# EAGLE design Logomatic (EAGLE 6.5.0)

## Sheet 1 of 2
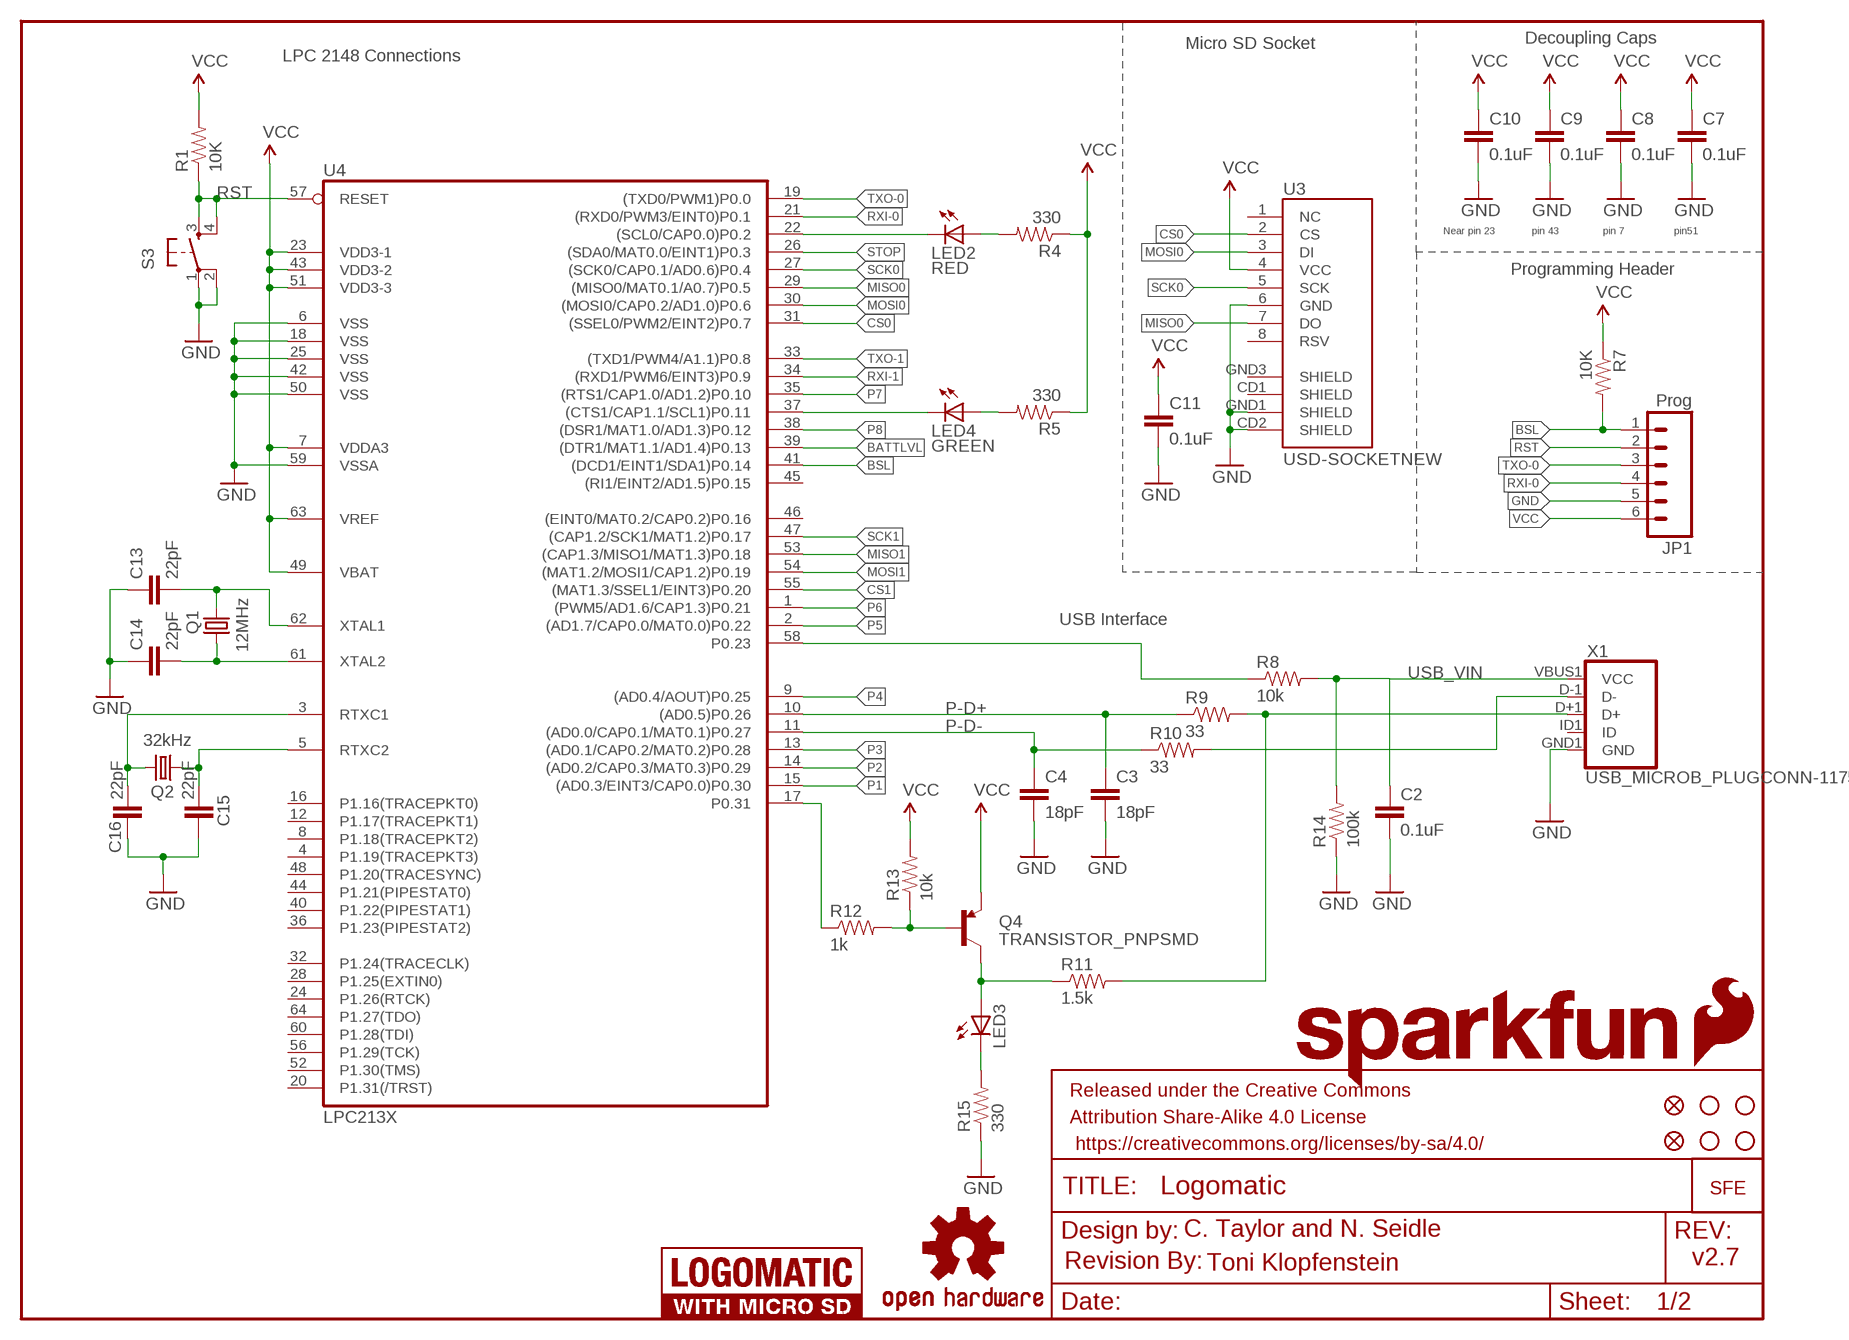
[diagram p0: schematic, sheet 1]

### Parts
C2  0.1uF  0.1UF-25V(+80/-20%)(0603)  [0603-CAP]
C3  18pF  18PF-50V-5%(0603)  [0603-CAP]
C4  18pF  18PF-50V-5%(0603)  [0603-CAP]
C7  0.1uF  0.1UF-25V(+80/-20%)(0603)  [0603-CAP]
C8  0.1uF  0.1UF-25V(+80/-20%)(0603)  [0603-CAP]
C9  0.1uF  0.1UF-25V(+80/-20%)(0603)  [0603-CAP]
C10  0.1uF  0.1UF-25V(+80/-20%)(0603)  [0603-CAP]
C11  0.1uF  0.1UF-25V(+80/-20%)(0603)  [0603-CAP]
C13  22pF  22PF-50V-5%(0603)  [0603-CAP]
C14  22pF  22PF-50V-5%(0603)  [0603-CAP]
C15  22pF  22PF-50V-5%(0603)  [0603-CAP]
C16  22pF  22PF-50V-5%(0603)  [0603-CAP]
FRAME2  FRAME-LETTER  [CREATIVE_COMMONS]
JP1  Prog  M06SIP  [1X06]
LED2  RED  LED-RED0603  [LED-0603]
LED3  LED-RED0603  [LED-0603]
LED4  GREEN  LED-GREEN0603  [LED-0603]
LOGO1  OSHW-LOGOL  [OSHW-LOGO-L]
LOGO2  SFE_LOGO_NAME.1_INCH  [SFE_LOGO_NAME_.1]
LOGO3  SFE_LOGO_FLAME.4_INCH  [SFE_LOGO_FLAME_.4]
Q1  12MHz  CRYSTAL5X3  [CRYSTAL-SMD-5X3]
Q2  32kHz  CRYSTAL32-SMD  [CRYSTAL-32KHZ-SMD]
Q4  TRANSISTOR_PNPSMD  [SOT23-3]
R1  10K  10KOHM1/10W1%(0603)0603  [0603-RES]
R4  330  330OHM1/10W1%(0603)  [0603-RES]
R5  330  330OHM1/10W1%(0603)  [0603-RES]
R7  10K  10KOHM1/10W1%(0603)0603  [0603-RES]
R8  10k  10KOHM1/10W1%(0603)0603  [0603-RES]
R9  33  33OHM1/10W1%(0603)  [0603]
R10  33  33OHM1/10W1%(0603)  [0603]
R11  1.5k  1.5KOHM1/10W1%(0603)  [0603]
R12  1k  1KOHM1/10W1%(0603)  [0603-RES]
R13  10k  10KOHM1/10W1%(0603)0603  [0603-RES]
R14  100k  100KOHM1/10W1%(0603)  [0603-RES]
R15  330  330OHM1/10W1%(0603)  [0603-RES]
S3  Reset  TAC_SWITCHSND  [TACTILE_SWITCH_SMD]
U3  USD-SOCKETNEW  [MICRO-SD-SOCKET-PP]
U4  LPC213X  [SQFP-S-10X10-64]
U$1  FIDUCIAL1X2  [FIDUCIAL-1X2]
U$2  FIDUCIAL1X2  [FIDUCIAL-1X2]
U$3  STAND-OFF  [STAND-OFF]
U$4  STAND-OFF  [STAND-OFF]
U$5  STAND-OFF  [STAND-OFF]
U$6  LOGOMATIC_LOGO  [LOGOMATIC_LOGO]
U$7  LOGO-SFESK  [SFE-LOGO-FLAME]
U$8  STAND-OFF  [STAND-OFF]
U$10  REVISION  [REVISION]
X1  USB_MICROB_PLUGCONN-11752  [USB-B-MICRO-SMD_V03]

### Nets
BATTLVL: U4.39((DTR1/MAT1.1/AD1.4)P0.13) ; also sheet 2
BSL: JP1.1 R7.2 U4.41((DCD1/EINT1/SDA1)P0.14)
CS0: U3.2(CS) U4.31((SSEL0/PWM2/EINT2)P0.7)
CS1: U4.55((MAT1.3/SSEL1/EINT3)P0.20) ; also sheet 2
GND [power]: C2.2 C3.2 C4.2 C7.2 C8.2 C9.2 C10.2 C11.2 C13.1 C14.1 C15.1 C16.1 JP1.5 R14.1 R15.1 S3.1 S3.2 U3.6(GND) U3.CD2(SHIELD) U3.GND1(SHIELD) U4.6(VSS) U4.18(VSS) U4.25(VSS) U4.42(VSS) U4.50(VSS) U4.59(VSSA) X1.GND1(GND) ; also sheet 2
MISO0: U3.7(DO) U4.29((MISO0/MAT0.1/A0.7)P0.5)
MISO1: U4.53((CAP1.3/MISO1/MAT1.3)P0.18) ; also sheet 2
MOSI0: U3.3(DI) U4.30((MOSI0/CAP0.2/AD1.0)P0.6)
MOSI1: U4.54((MAT1.2/MOSI1/CAP1.2)P0.19) ; also sheet 2
N$5: C13.2 Q1.3 U4.62(XTAL1)
N$6: C16.2 Q2.X2 U4.3(RTXC1)
N$7: LED2.A R4.2
N$9: C15.2 Q2.X1 U4.5(RTXC2)
N$16: R8.1 U4.58(P0.23)
N$17: Q4.1(B) R12.2 R13.1
N$19: LED4.A R5.2
N$21: C14.2 Q1.1 U4.61(XTAL2)
N$31: R12.1 U4.17(P0.31)
N$33: LED3.C R15.2
P1: U4.15((AD0.3/EINT3/CAP0.0)P0.30) ; also sheet 2
P2: U4.14((AD0.2/CAP0.3/MAT0.3)P0.29) ; also sheet 2
P3: U4.13((AD0.1/CAP0.2/MAT0.2)P0.28) ; also sheet 2
P4: U4.9((AD0.4/AOUT)P0.25) ; also sheet 2
P5: U4.2((AD1.7/CAP0.0/MAT0.0)P0.22) ; also sheet 2
P6: U4.1((PWM5/AD1.6/CAP1.3)P0.21) ; also sheet 2
P7: U4.35((RTS1/CAP1.0/AD1.2)P0.10) ; also sheet 2
P8: U4.38((DSR1/MAT1.0/AD1.3)P0.12) ; also sheet 2
P-D+: C3.1 R9.1 U4.10((AD0.5)P0.26)
P-D-: C4.1 R10.1 U4.11((AD0.0/CAP0.1/MAT0.1)P0.27)
RST: JP1.2 R1.1 S3.3 S3.4 U4.57(RESET)
RXI-0: JP1.4 U4.21((RXD0/PWM3/EINT0)P0.1)
RXI-1: U4.34((RXD1/PWM6/EINT3)P0.9) ; also sheet 2
SCK0: U3.5(SCK) U4.27((SCK0/CAP0.1/AD0.6)P0.4)
SCK1: U4.47((CAP1.2/SCK1/MAT1.2)P0.17) ; also sheet 2
STAT: LED3.A Q4.3(C) R11.1
STAT0: LED2.C U4.22((SCL0/CAP0.0)P0.2)
STAT1: LED4.C U4.37((CTS1/CAP1.1/SCL1)P0.11)
STOP: U4.26((SDA0/MAT0.0/EINT1)P0.3) ; also sheet 2
TXO-0: JP1.3 U4.19((TXD0/PWM1)P0.0)
TXO-1: U4.33((TXD1/PWM4/A1.1)P0.8) ; also sheet 2
USB_D+: R9.2 R11.2 X1.D+1(D+)
USB_D-: R10.2 X1.D-1(D-)
USB_VIN: C2.1 R8.2 R14.2 X1.VBUS1(VCC) ; also sheet 2
VCC: C7.1 C8.1 C9.1 C10.1 C11.1 JP1.6 Q4.2(E) R1.2 R4.1 R5.1 R7.1 R13.2 U3.4(VCC) U4.7(VDDA3) U4.23(VDD3-1) U4.43(VDD3-2) U4.49(VBAT) U4.51(VDD3-3) U4.63(VREF) ; also sheet 2
Unconnected: U3.1(NC) U3.8(RSV) U3.CD1(SHIELD) U3.GND3(SHIELD) U4.4(P1.19(TRACEPKT3)) U4.8(P1.18(TRACEPKT2)) U4.12(P1.17(TRACEPKT1)) U4.16(P1.16(TRACEPKT0)) U4.20(P1.31(/TRST)) U4.24(P1.26(RTCK)) U4.28(P1.25(EXTIN0)) U4.32(P1.24(TRACECLK)) U4.36(P1.23(PIPESTAT2)) U4.40(P1.22(PIPESTAT1)) U4.44(P1.21(PIPESTAT0)) U4.45((RI1/EINT2/AD1.5)P0.15) U4.46((EINT0/MAT0.2/CAP0.2)P0.16) U4.48(P1.20(TRACESYNC)) U4.52(P1.30(TMS)) U4.56(P1.29(TCK)) U4.60(P1.28(TDI)) U4.64(P1.27(TDO)) X1.ID1(ID)

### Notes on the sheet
- Decoupling Caps
- Micro SD Socket
- LPC 2148 Connections
- Near pin 23 | pin 43 | pin 7 | pin51
- Programming Header
- USB Interface
- C. Taylor and N. Seidle
- Toni Klopfenstein | v2.7

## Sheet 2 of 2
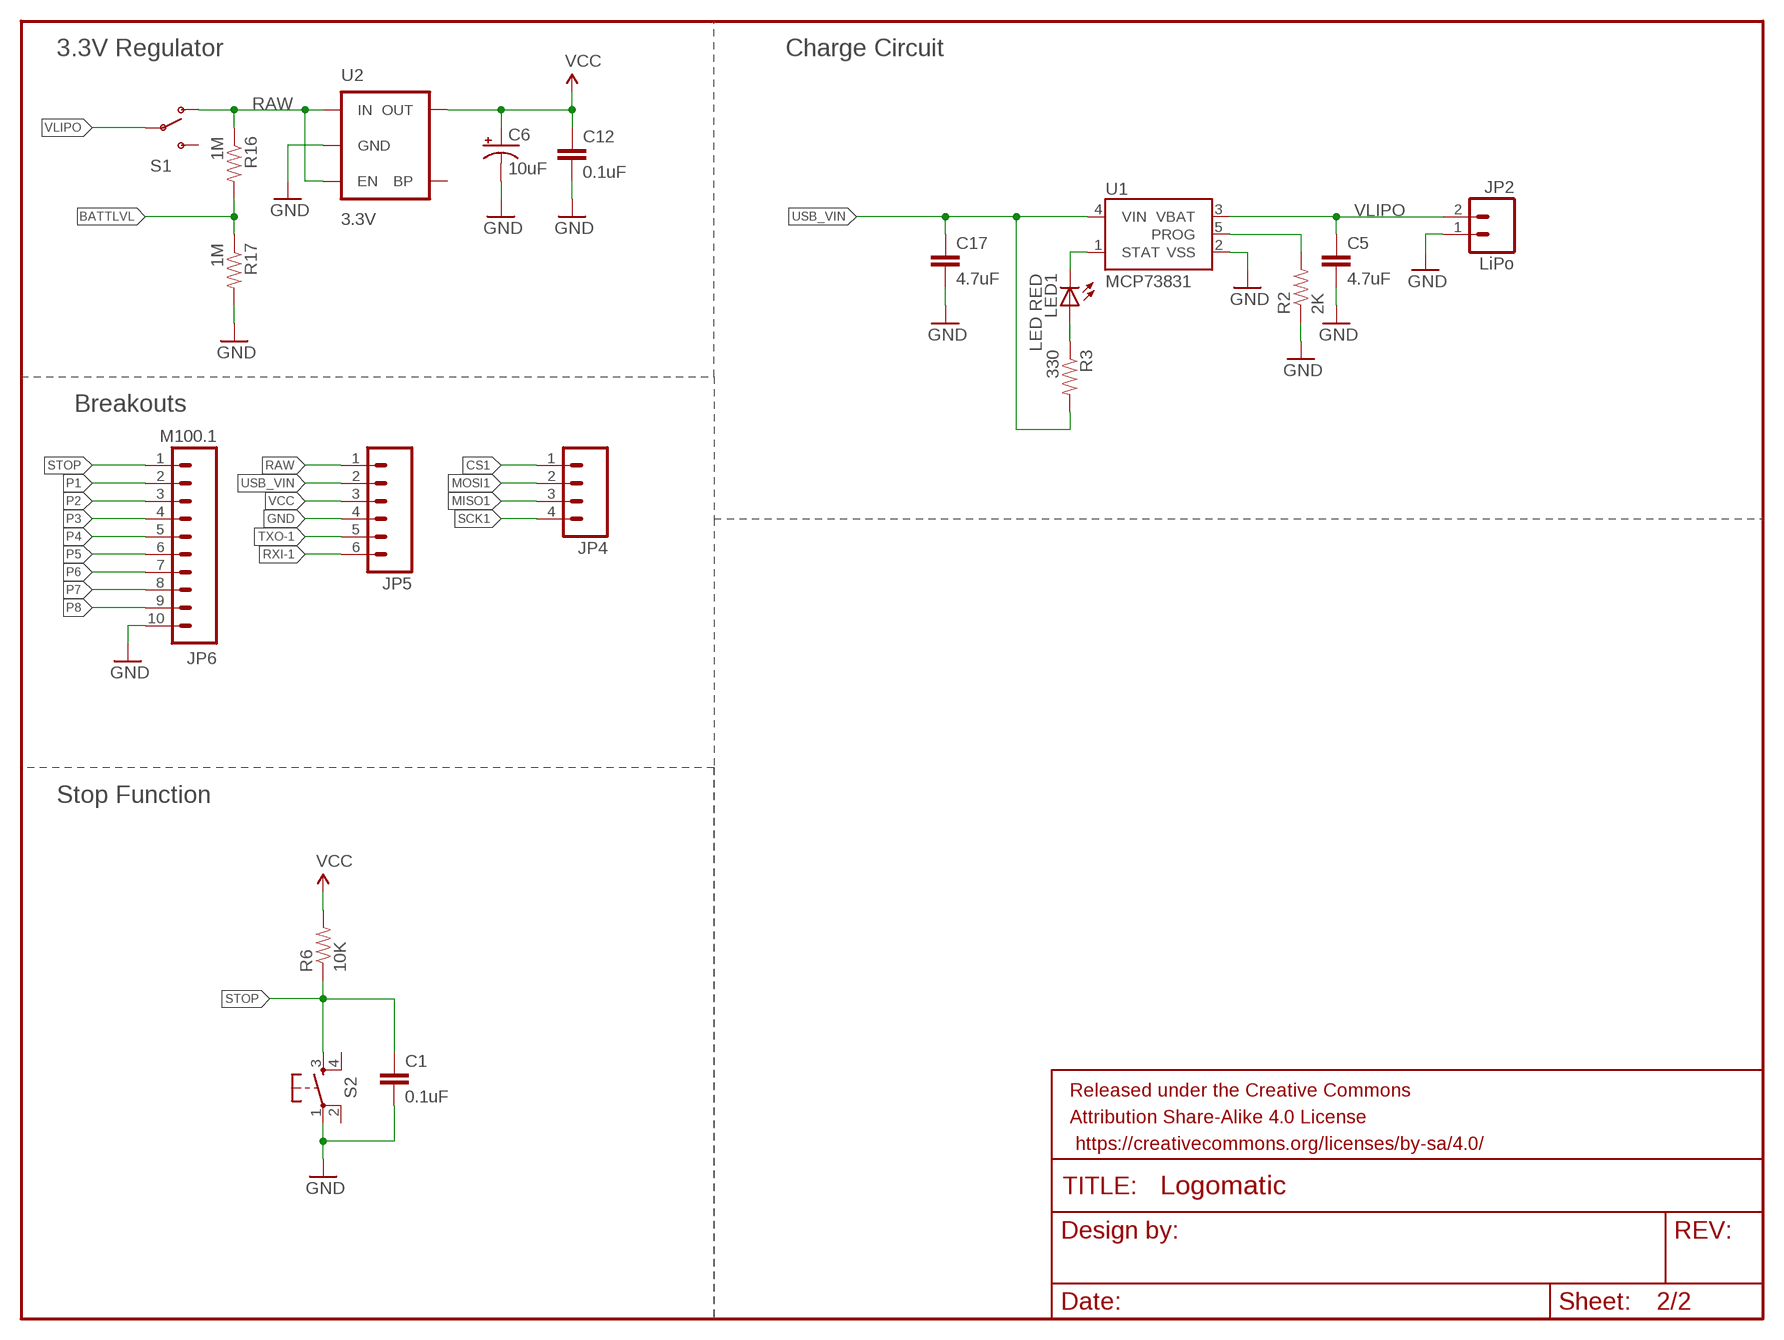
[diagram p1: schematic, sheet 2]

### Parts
C1  0.1uF  0.1UF-25V(+80/-20%)(0603)  [0603-CAP]
C5  4.7uF  4.7UF-6.3V-10%(0603)0603  [0603-CAP]
C6  10uF  10UF-16V-10%(TANT)  [EIA3216]
C12  0.1uF  0.1UF-25V(+80/-20%)(0603)  [0603-CAP]
C17  4.7uF  4.7UF-6.3V-10%(0603)0603  [0603-CAP]
FRAME4  FRAME-LETTER  [CREATIVE_COMMONS]
JP2  LiPo  M02-JST-2MM-SMT  [JST-2-SMD]
JP4  M04PTH  [1X04]
JP5  M06SIP  [1X06]
JP6  M100.1  M10"  [1X10]
LED1  LED RED  LED-RED0603  [LED-0603]
R2  2K  2.0KOHM1/10W5%(0603)  [0603-RES]
R3  330  330OHM1/10W1%(0603)  [0603-RES]
R6  10K  10KOHM1/10W1%(0603)0603  [0603-RES]
R16  1M  1MOHM1/10W1%(0603)  [0603-RES]
R17  1M  1MOHM1/10W1%(0603)  [0603-RES]
S1  SWITCH-SPSTSMD  [AYZ0202]
S2  Stop  TAC_SWITCHSND  [TACTILE_SWITCH_SMD]
U1  MCP73831  MCP73831SMD  [SOT23-5]
U2  3.3V  V_REG_LDOSMD  [SOT23-5]

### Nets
BATTLVL: R16.2 R17.1 ; also sheet 1
CS1: JP4.1 ; also sheet 1
GND [power]: C1.2 C5.2 C6.C(-) C12.2 C17.2 JP2.1 JP5.4 JP6.10 R2.1 R17.2 S2.1 U1.2(VSS) U2.2(GND) ; also sheet 1
MISO1: JP4.3 ; also sheet 1
MOSI1: JP4.2 ; also sheet 1
N$1: R2.2 U1.5(PROG)
N$12: LED1.C U1.1(STAT)
N$13: LED1.A R3.1
P1: JP6.2 ; also sheet 1
P2: JP6.3 ; also sheet 1
P3: JP6.4 ; also sheet 1
P4: JP6.5 ; also sheet 1
P5: JP6.6 ; also sheet 1
P6: JP6.7 ; also sheet 1
P7: JP6.8 ; also sheet 1
P8: JP6.9 ; also sheet 1
RAW: JP5.1 R16.1 S1.1(O) U2.1(IN) U2.3(EN)
RXI-1: JP5.6 ; also sheet 1
SCK1: JP4.4 ; also sheet 1
STOP: C1.1 JP6.1 R6.1 S2.3 ; also sheet 1
TXO-1: JP5.5 ; also sheet 1
USB_VIN: C17.1 JP5.2 R3.2 U1.4(VIN) ; also sheet 1
VCC: C6.A(+) C12.1 JP5.3 R6.2 U2.5(OUT) ; also sheet 1
VLIPO [power]: C5.1 JP2.2 S1.2(P) U1.3(VBAT)
Unconnected: S1.3(S) S2.2 S2.4 U2.4(BP)

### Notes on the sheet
- 3.3V Regulator | Charge Circuit
- Breakouts
- Stop Function

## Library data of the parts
C1 C2 C7-C12 = SparkFun-Capacitors:0.1UF-25V(+80/-20%)(0603): CAP-00810; PROD_ID: CAP-00810
C3 C4 = SparkFun-Capacitors:18PF-50V-5%(0603): CAP-08267; PROD_ID: CAP-08267
C5 C17 = SparkFun-Capacitors:4.7UF-6.3V-10%(0603): CAP-08280; PROD_ID: CAP-08280
C6 = SparkFun-Capacitors:10UF-16V-10%(TANT): CAP-00811; PROD_ID: CAP-00811
C13-C16 = SparkFun-Capacitors:22PF-50V-5%(0603): CAP-07876; PROD_ID: CAP-07876
FRAME2 FRAME4 = SparkFun-Aesthetics:FRAME-LETTER: Schematic Frame
JP1 JP5 = SparkFun:M06: Header 6 Standard 6-pin 0.1" header. Use with straight break away headers (SKU : PRT-00116), right angle break away headers (PRT-00553), swiss pins (PRT-00743), machine pins (PRT-00117), and female headers (PRT-00115). Molex polarized connector foot print use with SKU : PRT-08094 with associated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
JP2 = SparkFun:M02: Header 2
JP4 = SparkFun:M04: Header 4 Standard 4-pin 0.1" header. Use with straight break away headers (SKU : PRT-00116), right angle break away headers (PRT-00553), swiss pins (PRT-00743), machine pins (PRT-00117), and female headers (PRT-00115). Molex polarized connector foot print use with SKU : PRT-08231 with associated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
JP6 = SparkFun:M10: Header 10 Standard 10-pin 0.1" header. Use with straight break away headers (SKU : PRT-00116), right angle break away headers (PRT-00553), swiss pins (PRT-00743), machine pins (PRT-00117), and female headers (PRT-00115).
LED1 LED3 = SparkFun-LED:LED-RED: Assorted Red LEDs; PROD_ID: DIO-00819; VALUE: RED
LED2 = SparkFun-LED:LED-RED: Assorted Red LEDs; PROD_ID: DIO-00819
LED4 = SparkFun-LED:LED-GREEN: Various green LEDs; PROD_ID: DIO-00821
LOGO1 = SparkFun-Aesthetics:OSHW-LOGO: Open Source Hardware Logo This logo indicates the piece of hardware it is found on incorporates a OSHW license and/or adheres to the definition of open source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
LOGO2 = SparkFun-Aesthetics:SFE_LOGO_NAME: SFE Logo, name only
LOGO3 = SparkFun-Aesthetics:SFE_LOGO_FLAME: SFE Logo, flame only
Q1 = SparkFunEagle-6-6-07:CRYSTAL: Crystals
Q2 = SparkFun:CRYSTAL: Crystals
Q4 = SparkFun:TRANSISTOR_PNP
R1 R6 R7 = SparkFun-Resistors:10KOHM1/10W1%(0603): RES-00824; PROD_ID: RES-00824
R2 = SparkFun-Resistors:2.0KOHM1/10W5%(0603): RES-08296; PROD_ID: RES-08296; VALUE: 2.0k
R3-R5 R15 = SparkFun-Resistors:330OHM1/10W1%(0603): RES-00818; PROD_ID: RES-00818
R8 R13 = SparkFun-Resistors:10KOHM1/10W1%(0603): RES-00824; PROD_ID: RES-00824; VALUE: 10K
R9 R10 = SparkFun-Resistors:33OHM1/10W1%(0603): RES-08270; PROD_ID: RES-08270; VALUE: 33OHM
R11 = SparkFun-Resistors:1.5KOHM1/10W1%(0603): RES-08306; PROD_ID: RES-08306; VALUE: 1.5KOHM
R12 = SparkFun-Resistors:1KOHM1/10W1%(0603): RES-07856; PROD_ID: RES-07856; VALUE: 1K
R14 = SparkFun-Resistors:100KOHM1/10W1%(0603): RES-07828; PROD_ID: RES-07828
R16 R17 = SparkFun-Resistors:1MOHM1/10W1%(0603): RES-07868; PROD_ID: RES-07868
S1 = SparkFun:SWITCH-SPST: SPST Switch Simple slide switch. Spark Fun Electronics SKU : COM-00102
S2 S3 = SparkFunEagle-6-6-07:TAC_SWITCH: Momentary Switch Button commonly used for reset or general input. Spark Fun Electronics SKU : COM-00097
U1 = SparkFun:MCP73831
U2 = SparkFun:V_REG_LDO: Voltage Regulator LDO Standard 150mA LDO voltage regulator in SOT-23 layout. Micrel part MIC5205. BP (by-pass) pin is used to lower output noise with 470pF cap.
U3 = SparkFun-Connectors:USD-SOCKET: microSD Socket Push-push type uSD socket. Schematic element and footprint production proven. Spark Fun Electronics SKU : PRT-00127. tDoc lines correctly indicate media card edge positions when inserting (unlocked, locked, depressed).
U4 = SparkFun:LPC213X: LPC213x Schematic element and footprint for NXP LPC213x. Spark Fun Electronics SKU : COM-00520
U$1 U$2 = SparkFun:FIDUCIAL: Fiducial Alignment Points
U$3-U$5 U$8 = SparkFun:STAND-OFF: Stand Off
U$6 = SparkFun-Aesthetics:LOGOMATIC_LOGO: Logo for the Logomatic boards.
U$7 = SparkFun:LOGO-SFE: Spark Fun Electronics PCB Logo
U$10 = SparkFun-Aesthetics:REVISION
X1 = SparkFun-Connectors:USB_MICROB_PLUG: USB Micro-B Plug Comes in a variety of packages. Check out Hirose's ZX-x0 line: http://www.hirose.co.jp/cataloge_hp/e24200011.pdf; PROD_ID: CONN-11752

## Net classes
0 default: width 0.178 mm
1 power: width 0.203 mm
2 hv: width 0.254 mm, clearance 0.229 mm

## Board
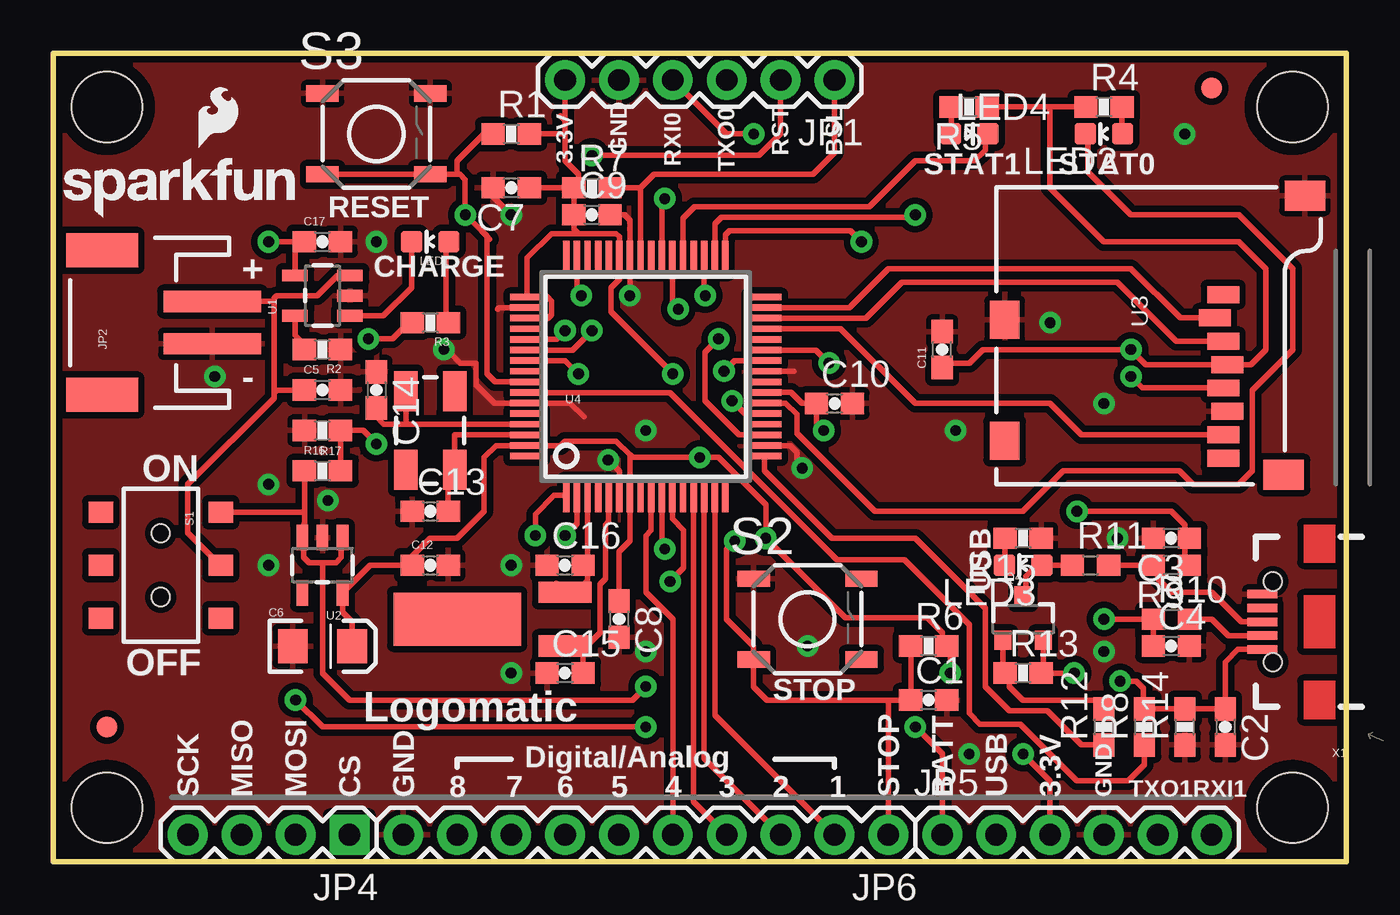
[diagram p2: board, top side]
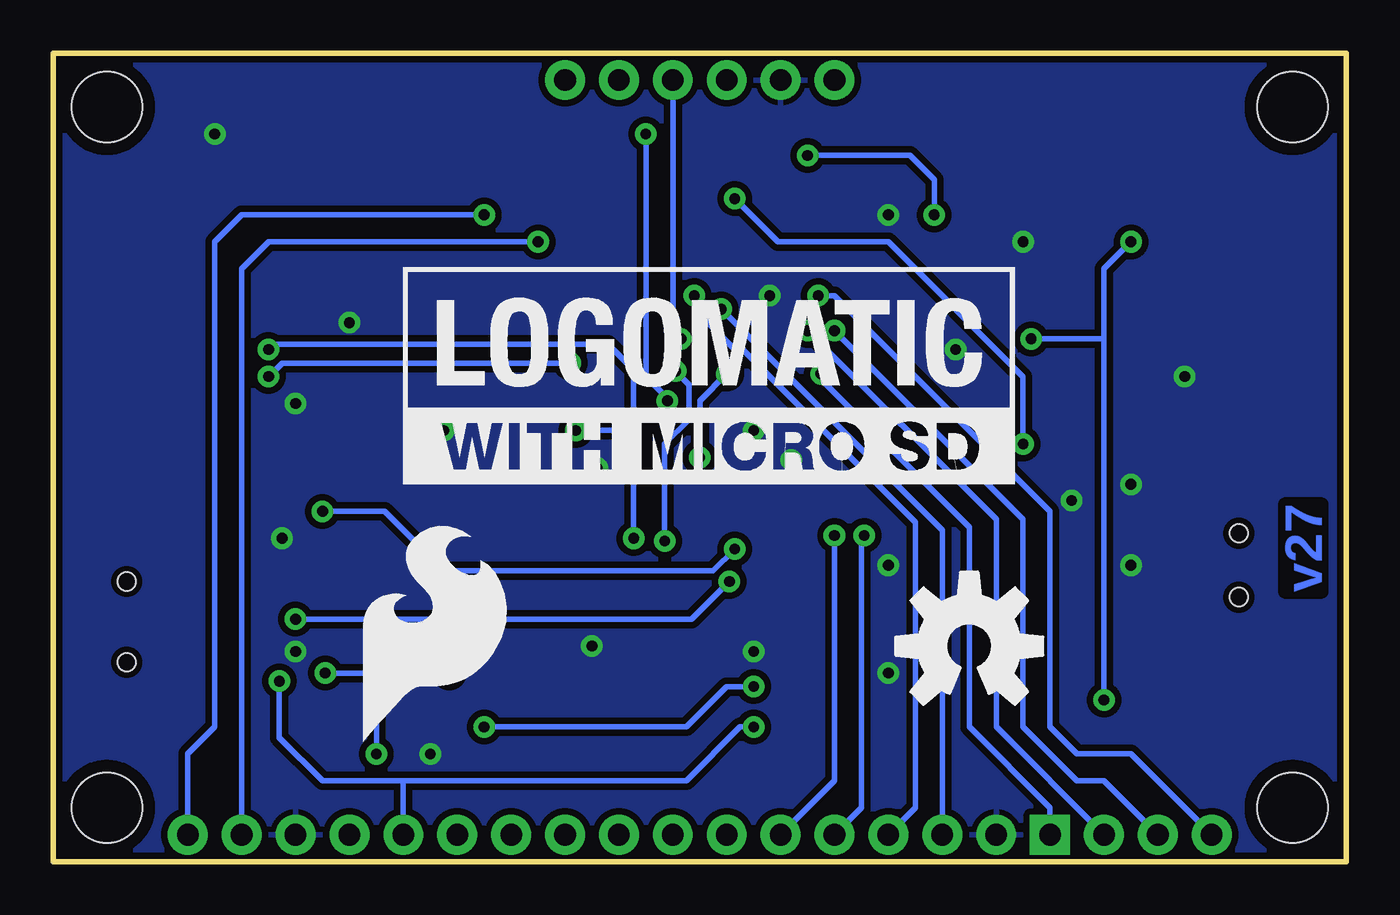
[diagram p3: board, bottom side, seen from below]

Size 60.96 x 38.1 mm. Coordinates in mm from the lower left corner, seen from the top.
Outline: 0,0 60.96,0 60.96,38.1 0,38.1 0,0
Copper layers (1*16): Top 0.035mm / dielectric 1.5mm / Bottom 0.035mm
Design rules "SparkFun *": minimum track width 8mil, minimum drill 20mil, track to track 8mil, track to pad 8mil, pad to pad 7mil, via to via 8mil, smd to smd 8mil, copper to edge 10mil, drill to drill 8mil, minimum pad ring 12mil, minimum via ring 10mil, stop-mask expansion 4mil, vias tented up to drill 20mil, thermal gap 10mil

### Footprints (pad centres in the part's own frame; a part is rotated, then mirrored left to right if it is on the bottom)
0603-CAP = smd 1.1 x 1: 1 -0.85,0; 2 0.85,0
EIA3216 = smd 1.4 x 1.6: A 1.4,0; C -1.4,0
1X06 = drill 1.016 pad 1.88: 1 0,0; 2 2.54,0; 3 5.08,0; 4 7.62,0; 5 10.16,0; 6 12.7,0
JST-2-SMD = smd 1 x 4.6: 1 -1,-3.7; 2 1,-3.7 | smd 1.6 x 3.4: NC1 -3.4,1.5; NC2 3.4,1.5
1X04 = drill 1.016 pad 1.88 square: 1 0,0 | drill 1.016 pad 1.88: 2 2.54,0; 3 5.08,0; 4 7.62,0
1X10 = drill 1.016 pad 1.88: 1 0,0; 2 2.54,0; 3 5.08,0; 4 7.62,0; 5 10.16,0; 6 12.7,0; 7 15.24,0; 8 17.78,0; 9 20.32,0; 10 22.86,0
LED-0603 = smd 1 x 1: A 0,-0.877; C 0,0.877
CRYSTAL-SMD-5X3 = smd 1.9 x 1.1: 1 -1.85,-1.15; 2 1.85,-1.15; 3 1.85,1.15; 4 -1.85,1.15
CRYSTAL-32KHZ-SMD = smd 2.5 x 6: SHEILD 0,5.08 | smd 1 x 2.5: X1 -1.27,0; X2 1.27,0
SOT23-3 = smd 0.8 x 0.9: 1 -0.95,-1; 2 0.95,-1; 3 0,1.1
0603-RES = smd 1.1 x 1: 1 -0.85,0; 2 0.85,0
0603 = smd 1.1 x 1: 1 -0.85,0; 2 0.85,0
AYZ0202 = smd 1 x 1.15: 1 -2.5,2.825; 2 0,2.825; 3 2.5,2.825; 4 -2.5,-2.825; 5 0,-2.825; 6 2.5,-2.825 | hole 0.85: 1.5,0; -1.5,0
TACTILE_SWITCH_SMD = smd 1.524 x 0.762: 1 -2.54,1.905; 2 2.54,1.905; 3 -2.54,-1.905; 4 2.54,-1.905
SOT23-5 = smd 0.55 x 1.2: 1 -0.95,-1.3; 2 0,-1.3; 3 0.95,-1.3; 4 0.95,1.3; 5 -0.95,1.3
MICRO-SD-SOCKET-PP = smd 0.8 x 1.5: 1 -8.94,10.7; 2 -7.84,10.3; 3 -6.74,10.7; 4 -5.64,10.9; 5 -4.54,10.7; 6 -3.44,10.9; 7 -2.34,10.7; 8 -1.24,10.7 | smd 1.8 x 1.4: CD1 -2.05,0.4; CD2 -7.75,0.4 | smd 1.4 x 1.9: GND1 -13.6,14.55; GND3 -0.45,13.55
SQFP-S-10X10-64 = smd 0.3 x 1.6: 1 -3.75,-5.6; 2 -3.25,-5.6; 3 -2.75,-5.6; 4 -2.25,-5.6; 5 -1.75,-5.6; 6 -1.25,-5.6; 7 -0.75,-5.6; 8 -0.25,-5.6; 9 0.25,-5.6; 10 0.75,-5.6; 11 1.25,-5.6; 12 1.75,-5.6; 13 2.25,-5.6; 14 2.75,-5.6; 15 3.25,-5.6; 16 3.75,-5.6; 33 3.75,5.6; 34 3.25,5.6; 35 2.75,5.6; 36 2.25,5.6; 37 1.75,5.6; 38 1.25,5.6; 39 0.75,5.6; 40 0.25,5.6; 41 -0.25,5.6; 42 -0.75,5.6; 43 -1.25,5.6; 44 -1.75,5.6; 45 -2.25,5.6; 46 -2.75,5.6; 47 -3.25,5.6; 48 -3.75,5.6 | smd 1.6 x 0.3: 17 5.6,-3.75; 18 5.6,-3.25; 19 5.6,-2.75; 20 5.6,-2.25; 21 5.6,-1.75; 22 5.6,-1.25; 23 5.6,-0.75; 24 5.6,-0.25; 25 5.6,0.25; 26 5.6,0.75; 27 5.6,1.25; 28 5.6,1.75; 29 5.6,2.25; 30 5.6,2.75; 31 5.6,3.25; 32 5.6,3.75; 49 -5.6,3.75; 50 -5.6,3.25; 51 -5.6,2.75; 52 -5.6,2.25; 53 -5.6,1.75; 54 -5.6,1.25; 55 -5.6,0.75; 56 -5.6,0.25; 57 -5.6,-0.25; 58 -5.6,-0.75; 59 -5.6,-1.25; 60 -5.6,-1.75; 61 -5.6,-2.25; 62 -5.6,-2.75; 63 -5.6,-3.25; 64 -5.6,-3.75
FIDUCIAL-1X2 = smd 1 x 1: 1 0,0
STAND-OFF = hole 3.302: 0,0
USB-B-MICRO-SMD_V03 = smd 1.4 x 0.4: D+1 2.7,0; D-1 2.7,0.65; GND1 2.7,-1.3; ID1 2.7,-0.65; VBUS1 2.7,1.3 | hole 0.85: 2.2,1.9; 2.2,-1.9

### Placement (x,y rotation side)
C1  41.27,7.62 0 top
C2  55.24,6.35 270 top
C3  52.7,15.24 180 top
C4  52.7,10.16 0 top
C5  12.7,22.23 0 top
C6  12.7,10.16 0 top
C7  21.59,31.75 180 top
C8  26.67,11.43 270 top
C9  25.4,30.48 0 top
C10  36.83,21.59 0 top
C11  41.91,24.13 90 top
C12  17.78,13.97 0 top
C13  17.78,16.51 0 top
C14  15.24,22.23 270 top
C15  24.13,8.89 0 top
C16  24.13,13.97 0 top
C17  12.7,29.21 0 top
FRAME2  not placed on the board
FRAME4  not placed on the board
JP1  36.83,36.83 180 top
JP2  3.81,25.4 90 top
JP4  13.97,1.27 180 top
JP5  41.91,1.27 0 top
JP6  39.37,1.27 180 top
LED1  17.78,29.21 90 top
LED2  49.53,34.29 90 top
LED3  45.72,13.97 90 top
LED4  43.18,34.29 270 top
LOGO1  17.78,10.16 0 bottom
LOGO2  0,29.84 0 top
LOGO3  46.99,5.08 0 bottom
Q1  17.78,20.32 270 top
Q2  24.13,11.43 90 top
Q4  45.72,11.43 0 top
R1  21.59,34.29 0 top
R2  12.7,24.13 180 top
R3  17.78,25.4 180 top
R4  49.53,35.56 0 top
R5  43.18,35.56 180 top
R6  41.27,10.16 0 top
R7  25.4,31.75 0 top
R8  51.44,6.35 90 top
R9  52.7,13.97 180 top
R10  52.7,11.43 0 top
R11  48.9,13.97 0 top
R12  49.53,6.35 90 top
R13  45.72,8.89 0 top
R14  53.34,6.35 90 top
R15  45.72,15.24 180 top
R16  12.7,18.41 0 top
R17  12.7,20.32 180 top
S1  5.08,13.97 270 top
S2  35.56,11.43 0 top
S3  15.24,34.29 0 top
U1  12.7,26.67 90 top
U2  12.7,13.97 180 top
U3  44.45,17.78 270 top
U4  27.94,22.86 0 top
U$1  2.54,6.35 0 top
U$2  54.61,36.45 0 top
U$3  2.54,2.54 0 top
U$4  58.42,2.54 0 top
U$5  2.54,35.56 0 top
U$6  44.45,17.78 0 bottom
U$7  6.86,33.66 0 top
U$8  58.42,35.56 0 top
U$10  not placed on the board
X1  59.69,11.3 180 top

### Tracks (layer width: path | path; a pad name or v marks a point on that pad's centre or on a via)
BATTLVL  (via drill 0.51)
  Top 0.254: U4.39 28.69,31.1 v28.83,31.24 | R16.2 R17.1 14.61,20.32 v15.24,19.68
  Bottom 0.254: v28.83,31.24 26.8,29.21 21.59,29.21 15.24,22.86 v15.24,19.68
BSL
  Top 0.254: U4.41 27.69,28.45 27.69,31.75 | JP1.1 36.83,33.4 35.81,32.38 28.32,32.38 27.69,31.75 | 27.69,31.75 R7.2
CS0
  Top 0.254: U4.31 37.54,26.11 39.37,27.94 50.8,27.94 53.12,25.62 U3.2
CS1  (via drill 0.51)
  Top 0.254: U4.55 24.14,23.61 v24.77,22.99
  Bottom 0.254: JP4.1 13.97,2.54 17.78,6.35 17.78,15.75 24.77,22.73 v24.77,22.99
GND  (via drill 0.51)
  Top 0.254: U4.25 34.92,23.11 | v27.18,26.67 27.19,26.68 U4.42 27.19,30.21 26.92,30.48 C9.2 26.04,30.48 | U4.6 26.69,18.39 26.42,18.67 | U4.18 34.75,19.61 35.05,19.3 35.05,18.8 v35.31,18.54 | 25.02,20.95 24.36,21.61 U4.59 20.81,21.61 19.94,22.48 19.94,23.5 19.18,23.5 18.8,23.88 | C7.2 20.74,31.33 v21.59,30.48 | U4.50 21.03,26.11 20.95,26.04
  other vias: 27.94,9.91 53.34,34.29 18.41,24.13 49.53,9.91 35.56,10.16 27.94,20.32 10.16,13.97 26.16,18.92 42.55,20.32 21.59,13.97 7.62,22.86 43.18,5.08 50.16,15.24 10.16,17.78 46.99,25.4 49.53,21.59 15.24,29.21 12.95,17.02 21.59,8.89
  pour Top (isolate 0.305): 0,0 60.96,0 60.96,38.1 0,38.1
  pour Bottom (isolate 0.305): 0,0 60.96,0 60.96,38.1 0,38.1
MISO0
  Top 0.254: U4.29 37.12,25.11 40.64,21.59 46.99,21.59 48.46,20.12 U3.7
MISO1  (via drill 0.51)
  Top 0.254: U4.53 23.72,24.61 v24.13,25.02
  Bottom 0.254: JP4.3 11.43,3.81 12.7,3.81 15.24,6.35 15.24,16.13 v24.13,25.02
MOSI0
  Top 0.254: U4.30 38.31,25.61 40.01,27.3 50.16,27.3 52.95,24.52 U3.3
MOSI1  (via drill 0.51)
  Top 0.254: U4.54 24.49,24.11 v25.4,25.02
  Bottom 0.254: JP4.2 16.51,6.35 16.51,16.13 v25.4,25.02
N$1
  Top 0.254: U1.5 11.4,24.8 12.05,24.14 11.87,24.14 R2.2
N$5
  Top 0.254: U4.62 18.92,20.11 18.92,20.07 18.93,20.06 Q1.3 18.63,18.17 C13.2
N$6
  Top 0.254: 25.19,13.76 U4.3 | 23.71,13.12 Q2.X2 24.64,12.7 25.19,13.25 25.19,13.76 | 25.19,13.76 C16.2
N$7
  Top 0.254: R4.2 50.38,34.32 LED2.A
N$9
  Top 0.254: U4.5 26.19,16.03 26.04,15.88 26.04,13.34 25.78,13.08 25.78,10.79 25.15,10.16 24.77,10.16 | 24.77,10.16 24.77,10.03 24.98,9.82 C15.2 | 24.77,10.16 Q2.X1
N$12
  Top 0.254: U1.1 15.56,25.72 16.89,27.05 16.89,29.2 LED1.C
N$13
  Top 0.254: R3.1 18.53,25.5 18.53,29.08 LED1.A
N$16
  Top 0.254: U4.58 22.35,22.1 29.08,22.1 36.96,14.22 40.13,14.22 43.18,11.18 43.18,6.99 43.69,6.48 45.59,6.48 48.26,3.81 50.67,3.81 51.44,4.57 R8.1
N$17
  Top 0.254: 49.49,7.24 R12.2 49.11,7.62 45.72,7.62 45.09,8.26 45.09,8.89 R13.1 44.77,8.99 Q4.1
N$19
  Top 0.254: R5.2 42.33,34.32 LED4.A
N$21
  Top 0.254: C14.2 15.24,20.95 15.59,20.61 16.64,20.61 | 16.64,20.61 U4.61 | 16.64,20.61 16.64,20.7 16.63,20.71 Q1.1
N$31
  Top 0.254: U4.17 33.54,19.06 33.53,19.05 33.53,18.41 36.7,15.24 40.64,15.24 43.94,11.94 43.94,8.26 45.09,7.11 46.86,7.11 48.48,5.5 R12.1
N$33
  Top 0.254: R15.2 44.87,14 LED3.C
P1
  Top 0.254: U4.15 31.19,6.91 JP6.2
P2
  Top 0.254: 30.69,17.36 U4.14 30.69,4.87 JP6.3
P3
  Top 0.254: U4.13 30.19,2.83 JP6.4
P4
  Top 0.254: U4.9 28.19,15.62 27.94,15.37 27.94,12.7 29.21,11.43 JP6.5
P5  (via drill 0.51)
  Top 0.254: U4.2 24.69,15.93 v24.13,15.37
  Bottom 0.254: v24.13,15.37 24.13,3.81 JP6.6
P6  (via drill 0.51)
  Top 0.254: 24.18,17.27 U4.1 23.61,17.26 22.73,16.38 v22.73,15.37
  Bottom 0.254: v22.73,15.37 22.86,15.24 22.86,2.54 JP6.7
P7  (via drill 0.51)
  Top 0.254: 30.69,28.49 U4.35 30.69,26.71 v30.73,26.67
  Bottom 0.254: v30.73,26.67 30.73,26.04 28.83,24.13 28.45,24.13 20.32,16 20.32,2.54 JP6.8
P8  (via drill 0.51)
  Top 0.254: U4.38 29.19,26.31 v29.46,26.04
  Bottom 0.254: JP6.9 19.05,15.62 v29.46,26.04
P-D+  (via drill 0.51)
  Top 0.254: U4.10 28.69,14.87 v28.83,14.73 | v48.26,16.51 52.7,16.51 53.34,15.88 53.34,15.46 C3.1 53.34,15.03 53.34,13.97 R9.1
  Bottom 0.254: v48.26,16.51 45.34,16.51 42.55,13.72 29.84,13.72 v28.83,14.73
P-D-  (via drill 0.51)
  Top 0.254: U4.11 29.19,16.15 29.72,15.62 29.72,13.84 v29.08,13.21 | v49.53,11.43 R10.1 C4.1
  Bottom 0.254: v49.53,11.43 30.86,11.43 v29.08,13.21
RAW  (via drill 0.51)
  Top 0.254: 11.75,15.55 U2.3 | 12.7,14.1 12.7,8.89 13.97,7.62 27.3,7.62 v27.94,8.26 | JP5.1 41.91,5.08 v40.64,6.35 | S1.1 11.81,16.47 11.85,16.51 | U2.3 11.81,15.33 11.81,15.88 11.85,15.91 11.85,16.51 | R16.1 11.85,16.51 | 12.7,14.1 12.06,14.1 11.81,14.35 11.81,15.21 U2.3 | 12.7,14.1 13.34,14.1 13.59,14.35 13.59,15.21 | 13.59,15.21 U2.1 | 13.59,15.21 13.59,15.49 13.65,15.55
  Bottom 0.254: v40.64,6.35 31.11,6.35 29.21,8.26 v27.94,8.26
RST  (via drill 0.51)
  Top 0.254: U4.57 22.1,22.61 20.83,22.61 20.45,22.99 20.45,29.46 | v25.4,33.27 33.27,33.27 34.29,34.29 JP1.2 | S3.3 S3.4 19.05,32.38 | 19.05,32.38 19.18,32.38 19.43,32.13 v19.43,30.48 20.19,29.72 20.45,29.46 | R1.1 20.32,34.29 19.05,33.02 19.05,32.38 | 20.57,29.34 20.45,29.46
  Bottom 0.254: v25.4,33.27 20.57,33.27 19.43,32.13 v19.43,30.48
RXI-0  (via drill 0.51)
  Top 0.254: U4.21 32.61,21.11 v32,21.72 | v33.02,34.29 31.75,34.29 JP1.4
  Bottom 0.254: v32,21.72 32,21.84 33.02,22.86 v33.02,34.29
RXI-1  (via drill 0.51)
  Top 0.254: U4.34 31.19,30.05 31.5,30.35 40.51,30.35 v40.64,30.48
  Bottom 0.254: v40.64,30.48 52.07,30.48 53.34,29.21 53.34,6.35 54.61,5.08 JP5.6
SCK0  (via drill 0.51)
  Top 0.254: U4.27 35.96,24.11 v36.58,23.5 | U3.5 51.34,22.32 v50.8,22.86
  Bottom 0.254: v36.58,23.5 50.16,23.5 v50.8,22.86
SCK1  (via drill 0.51)
  Top 0.254: U4.47 24.69,26.87 v24.89,26.67
  Bottom 0.254: JP4.4 10.16,5.08 12.7,5.08 13.97,6.35 13.97,16.51 24.13,26.67 v24.89,26.67
STAT
  Top 0.254: Q4.3 45.72,12.57 45.85,12.7 45.85,13.46 46.35,13.97 LED3.A R11.1
STAT0
  Top 0.254: U4.22 34.52,21.61 35.05,21.08 35.05,20.19 38.73,16.51 45.72,16.51 47.62,18.41 53.09,18.41 53.72,17.78 55.88,17.78 56.52,18.41 56.52,22.23 58.42,24.13 58.42,27.94 55.88,30.48 50.8,30.48 48.77,32.51 48.77,34.17 LED2.C
STAT1
  Top 0.254: U4.37 29.69,30.32 30.23,30.86 38.48,30.86 40.64,33.02 43.43,33.02 43.94,33.53 43.94,34.17 LED4.C
STOP  (via drill 0.51)
  Top 0.254: U4.26 32.12,23.61 v31.62,23.11 | v32.13,15.11 31.75,14.73 31.75,11.43 33.02,10.16 S2.3 33.02,8.26 33.66,7.62 39.37,7.62 | 39.37,7.62 C1.1 R6.1 | JP6.1 39.37,7.62
  Bottom 0.254: v31.62,23.11 30.99,22.48 30.99,20.83 32.13,19.68 v32.13,15.11
TXO-0  (via drill 0.51)
  Top 0.254: U4.19 32.34,20.11 30.73,21.72 30.73,24 v31.37,24.64
  Bottom 0.254: JP1.3 31.75,25.02 v31.37,24.64
TXO-1  (via drill 0.51)
  Top 0.254: U4.33 31.69,29.53 31.88,29.72 37.59,29.72 v38.1,29.21
  Bottom 0.254: v38.1,29.21 50.8,29.21 52.07,27.94 JP5.5
USB_D+
  Top 0.254: 50.23,13.97 50.18,13.92 50.13,13.97 R11.2 R9.2 52.07,13.76 52.07,13.34 52.7,12.7 54.61,12.7 56.01,11.3 X1.D+1
USB_D-
  Top 0.254: X1.D-1 55.39,10.65 54.61,11.43 R10.2
USB_VIN  (via drill 0.51)
  Top 0.254: v27.94,6.35 12.7,6.35 v11.43,7.62 | v10.16,29.21 11.43,29.21 | 11.43,29.21 C17.1 | U1.4 11.4,29.18 11.43,29.21 | R3.2 16.76,25.4 16,24.64 v14.86,24.64 | C2.1 R14.2 R8.2 | R8.2 51.22,7.2 | 55.12,7.33 C2.1 | X1.VBUS1 55.85,10 55.24,9.4 C2.1 | R8.2 51.4,7.24 51.4,8.17 51.05,8.51 v50.29,8.51
  Bottom 0.254: 44.45,3.81 31.11,3.81 28.57,6.35 v27.94,6.35 | 44.45,3.81 48.26,3.81 50.29,5.84 v50.29,8.51 | 44.45,3.81 JP5.2 | v11.43,7.62 11.43,24.64 | 11.43,24.64 v14.86,24.64 | 11.43,24.64 11.43,27.94 v10.16,29.21
VCC  (via drill 0.51)
  Top 0.254: 24.75,31.73 24.77,31.75 R7.1 | 24.77,29.59 23.5,29.59 22.35,28.45 22.35,26.67 22.34,26.66 U4.49 23.3,26.61 23.5,26.42 23.5,25.78 23.32,25.61 U4.51 | 24.77,29.59 26.54,29.59 26.69,29.44 U4.43 26.69,27.45 26.29,27.05 26.29,25.91 v29.21,22.99 | U4.23 34.79,22.11 35.31,21.59 C10.1 35.98,20.66 v36.32,20.32 | v48.13,8.89 R13.2 46.67,8.99 Q4.2 | C8.1 26.67,14.61 27.19,15.12 U4.7 27.19,19.16 | 24.13,34.92 JP1.6 | 27.19,19.16 27.3,19.05 v30.48,19.05 31.37,19.05 33.59,16.83 v33.59,15.24 37.34,11.49 41.21,11.49 41.91,10.79 41.91,10.38 R6.2 42.29,9.99 v42.29,8.89 | 27.19,19.16 26.54,19.81 24.13,19.81 23.93,19.61 U4.63 20.88,19.61 20.32,19.05 20.32,16.51 19.05,15.24 17.78,15.24 16.93,14.39 C12.1 14.95,13.97 U2.5 13.65,11.75 14.1,11.3 C6.A | JP5.3 46.99,3.81 v45.72,5.08 | 46.99,35.56 R4.1 | 46.99,35.56 46.99,31.75 49.53,29.21 55.88,29.21 57.15,27.94 57.15,24.13 56.44,23.42 U3.4 51.51,23.42 v50.8,24.13 43.81,24.13 43.18,23.5 42.12,23.5 C11.1 | 46.99,35.56 R5.1 | 23.91,35.14 24.13,34.92 | R7.1 C9.1 24.55,29.81 24.77,29.59 | 24.13,34.92 24.13,34.29 | 24.13,34.29 24.13,33.02 24.77,32.38 24.77,31.96 R7.1 | C7.1 R7.1 | R1.2 24.13,34.29
  Bottom 0.254: v33.59,15.24 33.59,20.32 | v42.29,8.89 45.72,8.89 | 45.72,8.89 v48.13,8.89 | 33.59,20.32 v36.32,20.32 | 33.59,20.32 33.59,23.18 34.8,24.38 50.55,24.38 v50.8,24.13 | v30.48,19.05 30.48,21.72 v29.21,22.99 | 45.72,8.89 v45.72,5.08
VLIPO
  Top 0.254: S1.2 7.87,13.97 6.35,15.49 6.35,17.78 10.41,21.84 10.41,22.1 | U1.3 13.4,27.62 12.45,26.67 10.54,26.67 10.41,26.54 10.41,26.42 | 10.41,22.1 10.41,26.42 | JP2.2 10.4,26.4 10.41,26.42 | C5.1 10.54,22.23 10.41,22.1

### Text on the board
Bottom: v27
tPlace: 3.3V | GND | RXI0 | TXO0 | RST | BSL | STAT1 | STAT0 | RESET | CHARGE | + | - | ON | USB | OFF | STOP | Logomatic | Digital/Analog | SCK | MISO | MOSI | CS | GND | 8 | 7 | 6 | 5 | 4 | 3 | 2 | 1 | STOP | BATT | USB | 3.3V | GND | TXO1 | RXI1
tValues: Horizontal JST
tDocu: C. Taylor and N. Seidle | Toni Klopfenstein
